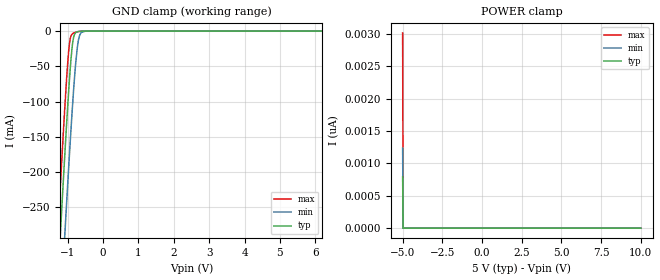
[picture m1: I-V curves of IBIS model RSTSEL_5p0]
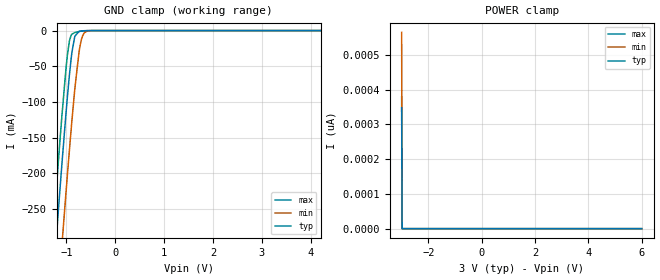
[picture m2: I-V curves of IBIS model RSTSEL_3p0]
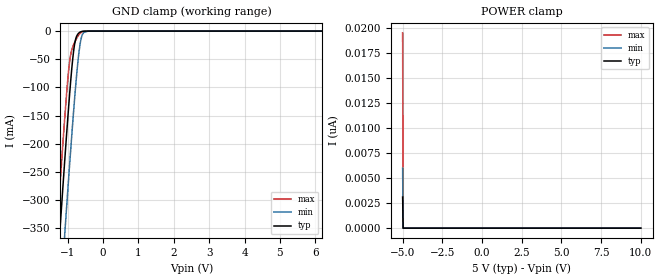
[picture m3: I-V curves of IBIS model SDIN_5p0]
|Texas Instruments Incorporated
|  part#   Digital Voltage Range
| DAC82002   2.7V - 5.5V
[IBIS Ver]   4.1
[File name]   dac82002.ibs
[File Rev]   1.0
[Date]   09/11/2022
[Source]
| Texas Instruments Incorporated.
| 12500 TI Blvd
| Dallas, TX -75243
[Notes]   Revision History:
| Rev 1.0: 09/11/2022
| - Initial version of the model
| - Model generated from simulations in TISPICE
| - C_comp although listed in numerical order of value are
|   obtained from varying PVT conditions. For PVT conditions for
|   each specific value refer the buffer description under
|   respective [Model]. IBIS model user is responsible for using
|   appropriate C_comp to simulate for Signal Integrity.
| - Warnings regarding combined Non-monotonicity of various models have been
|   reviewed and considered minor and can be ignored.
| - Model names with a trailing _3p0 contain the model for
|   3.0V operation. Model names with a trailing _5p0 contain the model
|   for 5.0V operation.
[Disclaimer]
| This model is designed as an aid for customers of Texas Instruments.
| TI and its licensors and suppliers make no warranties, either expressed
| or implied, with respect to this  model, including the warranties of
| merchantability or fitness for a particular purpose. The model is
| provided solely on an "as is" basis. The entire risk as to its quality
| and performance is with the customer.
| This model is subject to change without notice. Texas Instruments
| Incorporated is not responsible for updating this model.
[Copyright]
 (C) Copyright 2019 Texas Instruments Incorporated. All rights reserved.
|   Device
[Component]  DAC82002DRX | 10 pin VSON
[Manufacturer]   TI
[Package]
| variable   typ   min   max
R_pkg   0.05   0.04   0.06
L_pkg   1.0nH   0.8nH   1.2nH
C_pkg   0.2pF   0.16pF   0.24pF
[Pin]  signal_name   model_name   R_pin   L_pin   C_pin
1   VDD   POWER   na   na   na
2   VOUTA   NC   na   na   na
3   RSTSEL   RSTSEL   na   na   na
4   AGND   GND   na   na   na
5   RESET   RSTSEL   na   na   na
6   SCLK   SCLK   na   na   na
7   SYNCB   SCLK   na   na   na
8   SDIN   SDIN   na   na   na
9   VOUTB   NC   na   na   na
10   VREFIO   NC   na   na   na
|   Model Selectors
[Model Selector]  SDIN
SDIN_3p0  Input buffer at 3.0V operation
SDIN_5p0  Input buffer at 5.0V operation
[Model Selector]  SCLK
SCLK_3p0   input buffer at 3.0V operation
SCLK_5p0   input buffer at 5.0V operation
[Model Selector]  RSTSEL
RSTSEL_3p0   input buffer at 3.0V operation
RSTSEL_5p0   input buffer at 5.0V operation
| Models and submodels in the file (6): RSTSEL_5p0 (Input), RSTSEL_3p0 (Input), SDIN_5p0 (Input), SDIN_3p0 (Input), SCLK_5p0 (Input), SCLK_3p0 (Input)
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|   Model
[Model]   RSTSEL_5p0
Model_type   Input
Vinl = 1.5
Vinh = 3.5
|   typ   min   max
C_comp   0.423pF   0.377pF   0.481pF
[Voltage Range]   5   4.5   5.5
[Temperature Range]   25   125   -40
[Power Clamp Reference]   5   4.5   5.5
[GND Clamp Reference]   0   0   0
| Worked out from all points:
|   GND clamp passes 1 mA (typ) near -0.73 V on its own axis
[GND Clamp]
|   Voltage   I(typ)   I(min)   I(max)
-5V       -4.018A    -4.121A    -3.958A
-1.43V    -501.2mA   -615.9mA   -432.8mA
-1.25V    -331.9mA   -447mA     -263mA
-1.16V    -249.3mA   -364.1mA   -180.8mA
-1.085V   -182.4mA   -296.2mA   -115.2mA
-1.04V    -143.7mA   -256.2mA   -78.36mA
-950mV    -71.94mA   -178.6mA   -19.98mA
-875mV    -25.31mA   -118mA     -4.433mA
-800mV    -4.408mA   -64.17mA   -2.261mA
-680mV    -446.2uA   -10.05mA   -678.1uA
-500mV    -9.097uA   -173.1uA   -17.18uA
10V       0A         0A         0A
[POWER Clamp]
|   Voltage   I(typ)   I(min)   I(max)
-5V       793pA      1.236nA    3.013nA
-4.97V    0A         0A         0A
-4.955V   0A         0A         0A
10V       0A         0A         0A
|   Model
[Model]   RSTSEL_3p0
Model_type   Input
Vinl = 0.9
Vinh = 2.1
|   typ   min   max
C_comp   0.423pF   0.377pF   0.481pF
[Voltage Range]   3   2.7   3.3
[Temperature Range]   25   125   -40
[Power Clamp Reference]   3   2.7   3.3
[GND Clamp Reference]   0   0   0
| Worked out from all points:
|   GND clamp passes 1 mA (typ) near -0.73 V on its own axis
[GND Clamp]
|   Voltage   I(typ)   I(min)   I(max)
-3V       -2.035A    -2.143A    -1.972A
-1.281V   -360.7mA   -475.8mA   -291.9mA
-1.146V   -236.7mA   -351.3mA   -168.2mA
-1.092V   -188.6mA   -302.4mA   -121.1mA
-1.011V   -119.5mA   -230.8mA   -56.49mA
-939mV    -64.04mA   -169.5mA   -15.61mA
-885mV    -30.31mA   -125.8mA   -5.092mA
-831mV    -9.604mA   -85.27mA   -2.895mA
-705mV    -676.1uA   -16.7mA    -909.7uA
-642mV    -228.2uA   -4.238mA   -403.6uA
-552mV    -33.57uA   -536.7uA   -69.65uA
6V        0A         0A         0A
[POWER Clamp]
|   Voltage   I(typ)   I(min)   I(max)
-3V       347.9pA    564.7pA    379.3pA
-2.982V   0A         0A         0A
-2.973V   0A         0A         0A
6V        0A         0A         0A
|   Model
[Model]   SDIN_5p0
Model_type   Input
Vinl = 1.5
Vinh = 3.5
|   typ   min   max
C_comp   3.377pF   3.057pF   3.504pF
[Voltage Range]   5   4.5   5.5
[Temperature Range]   25   125   -40
[Power Clamp Reference]   5   4.5   5.5
[GND Clamp Reference]   0   0   0
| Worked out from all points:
|   GND clamp passes 1 mA (typ) near -0.61 V on its own axis
[GND Clamp]
|   Voltage   I(typ)   I(min)   I(max)
-5V       -4.075A    -4.197A    -4.003A
-1.43V    -557mA     -689.3mA   -477.9mA
-1.25V    -386.7mA   -519.1mA   -307.9mA
-1.145V   -289.5mA   -421.3mA   -211.9mA
-1.085V   -235.2mA   -366.1mA   -159.4mA
-1.055V   -208.5mA   -338.8mA   -134.2mA
-950mV    -119.3mA   -245mA     -59.1mA
-830mV    -36.45mA   -143.6mA   -24.41mA
-710mV    -5.467mA   -56.39mA   -9.431mA
-620mV    -1.144mA   -14.6mA    -2.617mA
-410mV    -5.32uA    -78.75uA   -6.596uA
10V       0A         0A         0A
[POWER Clamp]
|   Voltage   I(typ)   I(min)   I(max)
-5V       3.107nA    5.988nA    19.48nA
-4.97V    0A         0A         0A
-4.955V   0A         0A         0A
10V       0A         0A         0A
